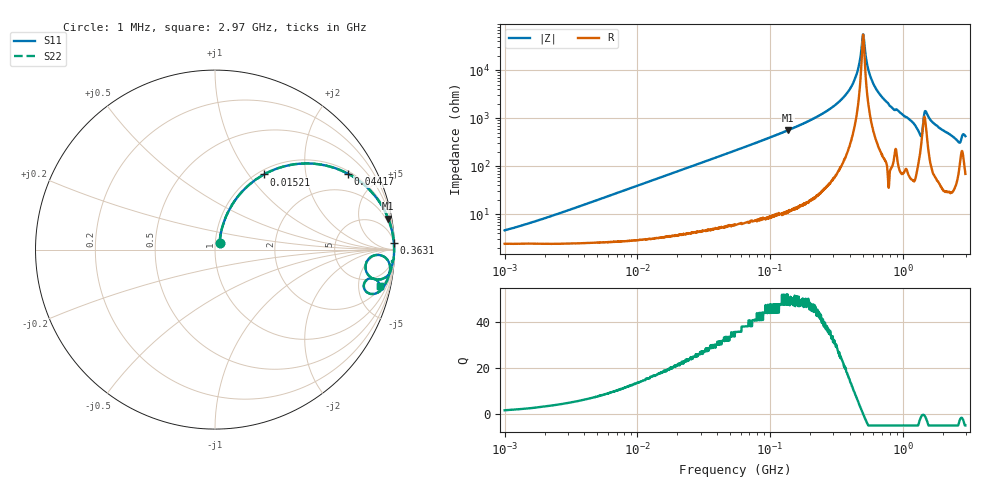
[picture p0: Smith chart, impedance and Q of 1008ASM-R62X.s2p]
!s-Parameter Generated by FASTRON Sdn. Bhd.
!FASTRON P/N : 1008ASM-R62X
!Keysight Technologies: E4991B_MY54100416_A.01.15
!Date: Tue Nov 21 09:26:41 2023
!Version  :Rev00  Wed Nov 22 15:16:34 2023
!Data & Calibration Information:
!Freq  S11  S21  S12  S22
!PortZ  Port1:50+j0  Port2:50+j0
!When reading reference impedance value at option line is always used.
! Remarks : This data is being provided solely for informational purposes.
# Hz S dB R 50
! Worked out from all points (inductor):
!   1599 points, 1 MHz to 2.97 GHz, reference 50 ohm
!   read as one part in series: L = 629 nH near 1.86 MHz
!   highest Q = 49.8 at 136.2 MHz (marker M1), where L = 652 nH
!   self-resonance near 502.7 MHz
!   S11 on the Smith chart (normalised r, x): 1 MHz: 1.05, +0.08; 15.21 MHz: 1.07, +1.19; 44.17 MHz: 1.11, +3.44; 363.1 MHz: 4, +57; 2.97 GHz: 2.39, -8.38
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1000000  -26.90 56.1  -0.22 -2.2  -0.22 -2.2  -26.90 56.1
3804036  -16.70 72.2  -0.31 -8.3  -0.31 -8.3  -16.70 72.2
1.439846e7  -6.37 58.1  -1.41 -28.6  -1.41 -28.6  -6.37 58.1
1.521322e7  -6.02 56.9  -1.53 -30.0  -1.53 -30.0  -6.02 56.9
4.416853e7  -1.38 29.7  -6.09 -58.5  -6.09 -58.5  -1.38 29.7
5.477226e7  -0.96 24.8  -7.54 -63.6  -7.54 -63.6  -0.96 24.8
1.361705e8  -0.17 10.1  -15.10 -78.8  -15.10 -78.8  -0.17 10.1
2.073156e8  -0.07 6.0  -19.60 -82.8  -19.60 -82.8  -0.07 6.0
3.631036e8  -0.02 2.0  -29.10 -85.2  -29.10 -85.2  -0.02 2.0
4.413523e8  -0.02 0.8  -37.00 -82.3  -37.00 -82.3  -0.02 0.8
4.66327e8  -0.02 0.5  -41.50 -77.5  -41.50 -77.5  -0.02 0.5
4.92715e8  -0.02 0.1  -50.60 -52.6  -50.60 -52.6  -0.02 0.1
5.051982e8  -0.02 -0.0  -54.90 9.7  -54.90 9.7  -0.02 -0.0
5.473095e8  -0.02 -0.5  -40.90 77.6  -40.90 77.6  -0.02 -0.5
5.870266e8  -0.02 -0.9  -35.60 82.3  -35.60 82.3  -0.02 -0.9
7.846996e8  -0.02 -3.0  -25.80 86.0  -25.80 86.0  -0.02 -3.0
1.147801e9  -0.11 -6.3  -19.20 80.2  -19.20 80.2  -0.11 -6.3
1.347129e9  -0.80 -10.5  -14.20 58.1  -14.20 58.1  -0.80 -10.5
1.496395e9  -0.32 -3.5  -23.10 57.1  -23.10 57.1  -0.32 -3.5
1.721456e9  -0.16 -7.2  -18.00 77.9  -18.00 77.9  -0.16 -7.2
2.594767e9  -0.74 -15.6  -11.30 65.0  -11.30 65.0  -0.74 -15.6
2.970126e9  -0.54 -12.6  -13.10 68.0  -13.10 68.0  -0.54 -12.6
